PROGRAM MAIN
VAR
	FB_GetUPSStatus: FB_GetUPSStatus;	
	dataloaded: BOOL;								//UPS数据文件读取状态（True为读取成功，False为读取失败）
	OldData: BOOL;									//UPS备份数据文件读取状态
	PersistentDataStatus: EPlcPersistentStatus;		//Persistent数据读取（恢复）状态
END_VAR
VAR PERSISTENT
	//设定的Persistent数据变量
	Int_persistent: INT;
	Float_persistent: LREAL;
	struct_persistent: dataDUT;
	Array_persistent: ARRAY[0..1048575] OF BYTE;
END_VAR

FB_GetUPSStatus(
	sNetId:= , 					//默认为本机Netid
	nPort:= , 					//ADS端口号，若不填写功能块会自动获取，默认0
	bEnable:= , 				//高电平有效，置True后循环读取UPS状态
	bValid=> , 					//当bValid为True时，stStatus的值有效
	bError=> , 
	nErrId=> , 
	stStatus=> );				//包含UPS信息的结构体
	

dataloaded:=_Appinfo.BootDataLoaded;
OldData:=_Appinfo.OldBootData;
PersistentDataStatus:=_Appinfo.PersistentStatus;

END_PROGRAM
